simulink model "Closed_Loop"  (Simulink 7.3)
settings: Solver=ode23s  StartTime=0.0  StopTime=100  MaxStep=0.01  RelTol=1e-3
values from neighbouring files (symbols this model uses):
  d2r = pi/180    (= 0.0174532925199)    [pl.m]    (also in run.m; Pl.m; start.m)
  J = [1045.3,  0,       19;      0,       641.02,  40;      19,      40,      505.05]    [run.m]    (also in start.m = [1.410986E+4, -0.3103E+2, -0.1187E+2;     -0.3103E+2,  1.304)
  npv = 28    [run.m]    (also in freq.m = 61)
undefined symbols (not defined in the file or in its folder): Au, Bu, Cu, Du

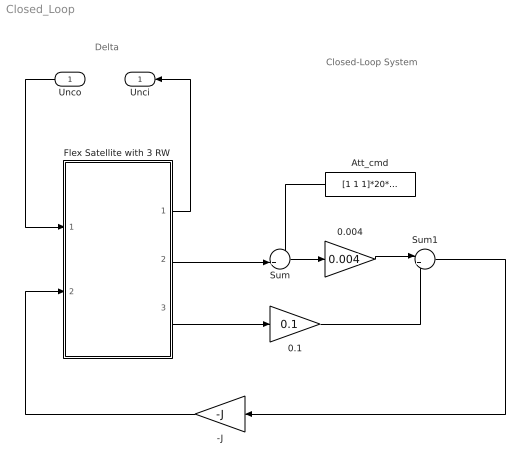
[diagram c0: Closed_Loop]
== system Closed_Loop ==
  note: Closed-Loop System
  note: Delta
  Unco : Inport  OutDataType=sfix(16)  OutScaling=2^0
  -J : Gain  Gain=-J  Multiplication=Matrix(K*u)  ParameterDataType=sfix(16)  ParameterScaling=2^0  OutDataType=sfix(16)  OutScaling=2^0
  0.004 : Gain  Gain=0.004  ParameterDataType=sfix(16)  ParameterScaling=2^0  OutDataType=sfix(16)  OutScaling=2^0
  0.1 : Gain  Gain=0.1  ParameterDataType=sfix(16)  ParameterScaling=2^0  OutDataType=sfix(16)  OutScaling=2^0
  Att_cmd : Constant  Value=[1 1 1]*20*d2r  OutDataType=sfix(16)  OutScaling=2^0
  Flex Satellite with 3 RW : Subsystem
  Sum : Sum  Inputs=-+|  OutDataType=sfix(16)  OutScaling=2^0
  Sum1 : Sum  Inputs=|++  OutDataType=sfix(16)  OutScaling=2^0
  Unci : Outport  OutDataType=sfix(16)  OutScaling=2^0
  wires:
  0.1/1 -> Sum1/2
  0.004/1 -> Sum1/1
  Sum/1 -> 0.004/1
  Att_cmd/1 -> Sum/1
  Flex Satellite with 3 RW/2(attit) -> Sum/2
  Flex Satellite with 3 RW/3(rate) -> 0.1/1
  Flex Satellite with 3 RW/1(Unci) -> Unci/1
  Unco/1 -> Flex Satellite with 3 RW/1(Unco)
  Sum1/1 -> -J/1
  -J/1 -> Flex Satellite with 3 RW/2(Trw)

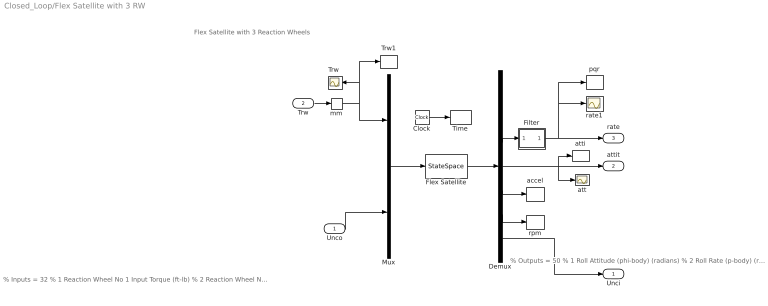
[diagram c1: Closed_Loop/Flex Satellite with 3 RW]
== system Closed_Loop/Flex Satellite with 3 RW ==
  note: Flex Satellite with 3 Reaction Wheels
  note: % Inputs = 32 % 1 Reaction Wheel No 1 Input Torque (ft-lb) % 2 Reaction Wheel No 2 Input Torque (ft-lb) % 3 Reaction Wheel No 3 Input Torque (ft-lb) % 4 Ext Torque Direct.=( 0.0000 1.0000 0.0000) Param Variations= 28 % 5 I_xx : 4.783 % Variation % 6 I_xx : 4.783 % Variation % 7 I_yy : 4.680 % Variation % 8 I_yy : 4.680 % Variation % 9 I_yy : 4.680 % Variation % 10 I_zz : 4.950 % Variation % 11 I_zz : 4.950 % Variation % 12 RWinert 1: 20.000 % Variation % 13 RW_H0 1: 0.2094E-01 Addit. Variat. % 14 RW_H0 1: 0.2094E-01 Addit. Variat. % 15 HDirect 1: 14.003 % Variation % 16 HDirect 1: 14.003 % Variation % 17 RWinert 2: 20.000 % Variation % 18 RW_H0 2: 0.2094E-01 Addit. Variat. % 19 RW_H0 2: 0.2094E-01 Addit. Variat. % 20 HDirect 2: 14.003 % Variation % 21 RWinert 3: 20.000 % Variation % 22 RW_H0 3: 0.2094E-01 Addit. Variat. % 23 RW_H0 3: 0.2094E-01 Addit. Variat. % 24 HDirect 3: 14.003 % Variation % 25 W_flex 1: 0.3000 Addit. Variat. % 26 W_flex 2: 0.4000 Addit. Variat. % 27 W_flex 3: 0.6000 Addit. Variat. % 28 W_flex 4: 2.000 Addit. Variat. % 29 W_flex 5: 2.000 Addit. Variat. % 30 W_flex 6: 10.00 Addit. Variat. % 31 W_flex 7: 10.00 Addit. Variat. % 32 W_flex 8: 10.00 Addit. Variat.
  note: % Outputs = 50 % 1 Roll Attitude (phi-body) (radians) % 2 Roll Rate (p-body) (rad/sec) % 3 Pitch Attitude (thet-bdy) (radians) % 4 Pitch Rate (q-body) (rad/sec) % 5 Yaw Attitude (psi-body) (radians) % 6 Yaw Rate (r-body) (rad/sec) % 7 Angle of attack, alfa, (radians) % 8 Angle of sideslip, beta, (radian) % 9 Change in Altitude, delta-h, (feet) % 10 Forward Acceleration (V-dot) (ft/sec) % 11 Cross Range Velocity (Vcr) (ft/sec) % 12 Rate-Gyro # 1, Roll Rate (Body) (rad/sec) % 13 Rate-Gyro # 2, Pitch Rate (Body) (rad/sec) % 14 Rate-Gyro # 3, Yaw Rate (Body) (rad/sec) % 15 Gyro # 4, Roll Attitude (Body) (radians) % 16 Gyro # 5, Pitch Attitude (Body) (radians) % 17 Gyro # 6, Yaw Attitude (Body) (radians) % 18 Accelerom # 1, (along X), (ft/sec^2) Translat. Acceler % 19 Accelerom # 2, (along Y), (ft/sec^2) Translat. Acceler % 20 Reaction Wheel # 1 Rate (rpm) relative to vehicle % 21 Reaction Wheel # 2 Rate (rpm) relative to vehicle % 22 Reaction Wheel # 3 Rate (rpm) relative to vehicle Param Variations= 28 % 23 I_xx : 4.783 % Variation % 24 I_xx : 4.783 % Variation % 25 I_yy : 4.680 % Variation % 26 I_yy : 4.680 % Variation % 27 I_yy : 4.680 % Variation % 28 I_zz : 4.950 % Variation % 29 I_zz : 4.950 % Variation % 30 RWinert 1: 20.000 % Variation % 31 RW_H0 1: 0.2094E-01 Addit. Variat. % 32 RW_H0 1: 0.2094E-01 Addit. Variat. % 33 HDirect 1: 14.003 % Variation % 34 HDirect 1: 14.003 % Variation % 35 RWinert 2: 20.000 % Variation % 36 RW_H0 2: 0.2094E-01 Addit. Variat. % 37 RW_H0 2: 0.2094E-01 Addit. Variat. % 38 HDirect 2: 14.003 % Variation % 39 RWinert 3: 20.000 % Variation % 40 RW_H0 3: 0.2094E-01 Addit. Variat. % 41 RW_H0 3: 0.2094E-01 Addit. Variat. % 42 HDirect 3: 14.003 % Variation % 43 W_flex 1: 0.3000 Addit. Variat. % 44 W_flex 2: 0.4000 Addit. Variat. % 45 W_flex 3: 0.6000 Addit. Variat. % 46 W_flex 4: 2.000 Addit. Variat. % 47 W_flex 5: 2.000 Addit. Variat. % 48 W_flex 6: 10.00 Addit. Variat. % 49 W_flex 7: 10.00 Addit. Variat. % 50 W_flex 8: 10.00 Addit. Variat.
  Unco : Inport  OutDataType=sfix(16)  OutScaling=2^0
  Trw : Inport  Port=2  OutDataType=sfix(16)  OutScaling=2^0
  Clock : Clock
  Demux : Demux  Outputs="[6, 5, 3, 3, 2, 3,  npv]"
  Filter : Subsystem
  Flex Satellite : StateSpace  A=Au  B=Bu  C=Cu  D=Du
  Mux : Mux  Inputs="[3, 1,  npv]"
  Time : ToWorkspace  VariableName=time  SampleTime=-1  SaveFormat=Array
  "Trw " : Scope
  Trw1 : ToWorkspace  VariableName=Trw  SampleTime=-1  SaveFormat=Array
  accel : ToWorkspace  VariableName=acc  SampleTime=-1  SaveFormat=Array
  att : Scope
  atti : ToWorkspace  VariableName=atti  SampleTime=-1  SaveFormat=Array
  mm : Memory
  pqr : ToWorkspace  VariableName=pqr  SampleTime=-1  SaveFormat=Array
  rate1 : Scope
  rpm : ToWorkspace  VariableName=rpm  SampleTime=-1  SaveFormat=Array
  Unci : Outport  OutDataType=sfix(16)  OutScaling=2^0
  attit : Outport  Port=2  OutDataType=sfix(16)  OutScaling=2^0
  rate : Outport  Port=3  OutDataType=sfix(16)  OutScaling=2^0
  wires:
  Demux/4 -> attit/1, att/1, atti/1
  Demux/3 -> Filter/1(In)
  Demux/5 -> accel/1
  Demux/6 -> rpm/1
  Mux/1 -> Flex Satellite/1
  Flex Satellite/1 -> Demux/1
  Demux/7 -> Unci/1
  Trw/1 -> mm/1
  Unco/1 -> Mux/3
  Filter/1(Ou) -> rate/1, rate1/1, pqr/1
  Clock/1 -> Time/1
  mm/1 -> Mux/1, "Trw "/1, Trw1/1

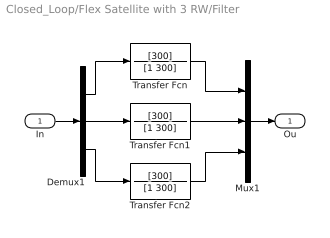
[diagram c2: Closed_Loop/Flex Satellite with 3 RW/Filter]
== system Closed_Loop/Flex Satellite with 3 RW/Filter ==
  In : Inport  OutDataType=sfix(16)  OutScaling=2^0
  Demux1 : Demux  Outputs=3
  Mux1 : Mux  Inputs=3
  Transfer Fcn : TransferFcn  Numerator=[300]  Denominator=[1 300]
  Transfer Fcn1 : TransferFcn  Numerator=[300]  Denominator=[1 300]
  Transfer Fcn2 : TransferFcn  Numerator=[300]  Denominator=[1 300]
  Ou : Outport  OutDataType=sfix(16)  OutScaling=2^0
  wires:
  Transfer Fcn1/1 -> Mux1/2
  Transfer Fcn/1 -> Mux1/1
  Transfer Fcn2/1 -> Mux1/3
  Demux1/2 -> Transfer Fcn1/1
  Demux1/1 -> Transfer Fcn/1
  Demux1/3 -> Transfer Fcn2/1
  In/1 -> Demux1/1
  Mux1/1 -> Ou/1
